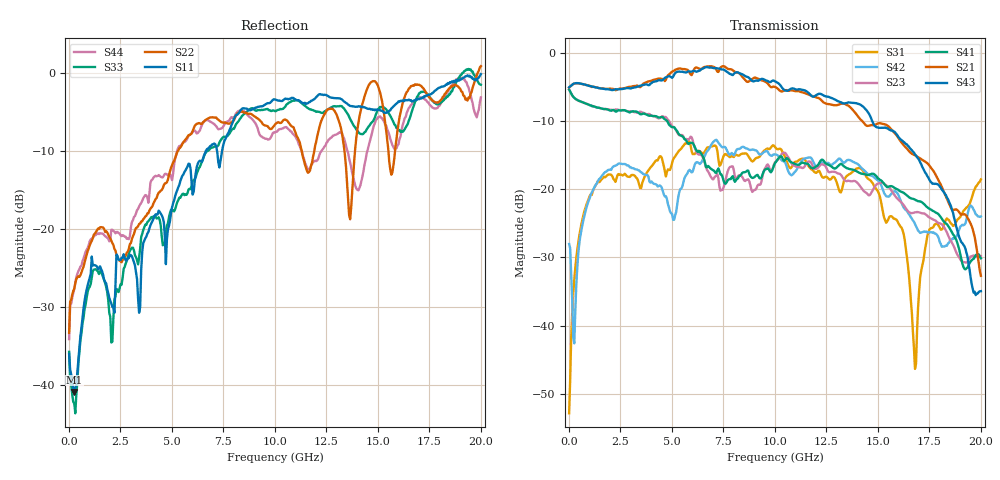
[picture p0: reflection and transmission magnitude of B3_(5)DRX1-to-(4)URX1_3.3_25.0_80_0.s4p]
!Agilent Technologies,N5225A,MY51451112,A.09.50.13
!Agilent N5225A: A.09.50.13
!Date: Sunday, March 12, 2017 05:20:40
!Correction: S11(Full 4 Port(1,2,3,4))
!S12(Full 4 Port(1,2,3,4))
!S13(Full 4 Port(1,2,3,4))
!S14(Full 4 Port(1,2,3,4))
!S21(Full 4 Port(1,2,3,4))
!S22(Full 4 Port(1,2,3,4))
!S23(Full 4 Port(1,2,3,4))
!S24(Full 4 Port(1,2,3,4))
!S31(Full 4 Port(1,2,3,4))
!S32(Full 4 Port(1,2,3,4))
!S33(Full 4 Port(1,2,3,4))
!S34(Full 4 Port(1,2,3,4))
!S41(Full 4 Port(1,2,3,4))
!S42(Full 4 Port(1,2,3,4))
!S43(Full 4 Port(1,2,3,4))
!S44(Full 4 Port(1,2,3,4))
!S4P File: Measurements: <S11,S12,S13,S14>,
!<S21,S22,S23,S24>,
!<S31,S32,S33,S34>,
!<S41,S42,S43,S44>:
# Hz S  dB  R 50
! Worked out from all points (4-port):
!   401 points, 10 MHz to 20 GHz, reference 50 ohm
!   strongest paths, dB at 10 MHz, 5.008 GHz, 10.01 GHz, 15 GHz, 20 GHz:
!     S43: -5.0, -3.6, -4.1, -10.9, -35.0
!     S21: -5.0, -2.7, -5.0, -10.3, -32.7
!     S41: -5.3, -10.9, -16.1, -18.4, -30.1
!     S23: -5.3, -10.7, -16.0, -19.1, -29.8
!     S42: -28.0, -23.6, -14.9, -18.7, -24.0
!     S31: -52.9, -16.1, -13.8, -20.3, -18.5
!   lowest |S11| = -40.9 dB at 259.9 MHz (marker M1), VSWR 1.02, Z = 50.3 - j0.859 ohm
!   |S11| at or under -10 dB: start of sweep to 6.654 GHz; 7.189 GHz to 7.437 GHz (248.6 MHz wide, 3.4 % of centre)
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1e7  -36.06 -39.0  -67.93 -157.6  -53.43 24.0  -62.27 106.2
     -5.02 1.2  -33.35 38.8  -5.33 179.8  -28.00 38.3
     -52.90 21.6  -68.83 92.2  -35.78 -45.5  -61.21 143.9
     -5.33 179.8  -28.02 37.5  -5.00 1.3  -34.16 45.3
2.59875e8  -40.92 -71.9  -49.77 56.7  -33.18 94.8  -50.25 53.8
           -4.45 -8.1  -27.69 -131.5  -6.55 162.0  -42.17 -161.2
           -33.26 95.2  -49.89 58.4  -42.40 -79.4  -50.39 55.4
           -6.55 161.2  -42.62 -171.3  -4.44 -8.9  -27.73 -137.4
5.257375e9  -15.07 83.7  -34.82 5.8  -14.68 30.1  -34.61 -7.2
            -2.32 173.3  -10.20 140.6  -11.64 -57.8  -22.50 71.9
            -14.70 28.4  -34.81 7.3  -16.60 101.5  -36.72 6.8
            -11.47 -75.4  -22.20 69.5  -2.72 162.8  -9.99 117.8
8.30585e9  -4.91 38.3  -39.40 -100.1  -14.95 -2.2  -36.58 -139.8
           -3.02 27.6  -5.01 79.7  -17.91 -133.6  -13.84 48.0
           -14.94 -2.3  -32.60 -123.6  -5.91 58.1  -32.03 -161.3
           -18.00 -155.6  -14.03 50.1  -2.97 14.6  -4.84 44.6
1.230385e10  -2.81 -20.1  -35.83 -162.6  -18.06 -23.7  -37.49 159.0
             -7.07 -135.5  -5.86 73.3  -16.31 81.3  -16.04 36.8
             -18.22 -22.4  -34.96 -152.4  -5.15 -9.2  -34.12 160.2
             -15.62 38.9  -16.07 38.7  -6.10 -162.3  -9.87 -7.0
1.68016e10  -3.56 -76.8  -35.62 110.4  -46.45 -64.8  -36.32 82.8
            -14.99 36.6  -1.50 70.1  -23.37 -157.5  -25.20 62.9
            -46.37 -92.9  -32.94 123.4  -3.76 -83.2  -33.49 80.8
            -21.50 152.7  -25.09 63.4  -14.86 -16.8  -3.49 -60.6
2e10  -0.19 -114.0  -33.06 62.9  -18.57 122.1  -35.49 21.2
      -32.70 -93.9  0.83 17.1  -29.79 55.3  -23.91 102.0
      -18.54 122.1  -33.93 40.0  -1.55 -87.6  -35.19 -7.9
      -30.12 18.1  -23.97 102.5  -34.96 -123.7  -3.17 -136.4
